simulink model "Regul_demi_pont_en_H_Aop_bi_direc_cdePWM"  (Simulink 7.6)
settings: Solver=ode15s  StartTime=0.0  StopTime=0.01  FixedStep=0.01  RelTol=1e-3
InitFcn:
  | clc
  | delete *.mat
  | close all
  | clear all
StopFcn:
  | close all, clc
  | load reg_vit.mat
  | 
  | plot(x(1,:),x(2,:),x(1,:),x(3,:))
  | xlabel('temps')
  | title('Consigne et vitesse angulaire - Moteur CC, 1/2 Pont en H bidirectionnel - Cde PWM')
  | grid
  | 
  | figure
  | load cde_PWM.mat
  | plot(u(1,:),u(2,:))
  | axis([0 4e-3 -0.5 5.5])
  | xlabel('temps')
  | title('Commande PWM')
  | grid
undefined symbols (not defined in the file or in its folder): sigbuilder_block
libraries: fl_lib x24, elec_lib x15, nesl_utility x15, simulink x1

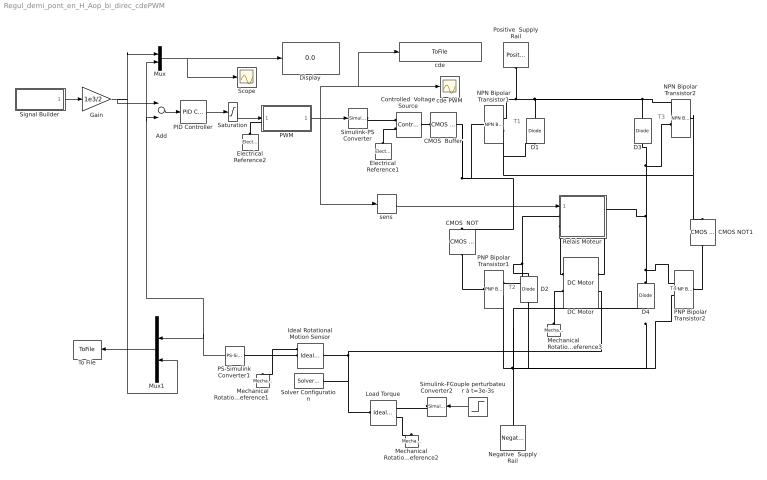
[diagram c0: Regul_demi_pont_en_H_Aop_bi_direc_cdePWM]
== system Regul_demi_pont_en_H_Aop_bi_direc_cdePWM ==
  note: T1
  note: T4
  note: T3
  note: T2
  Add : Sum  Inputs=+-
  CMOS  Buffer : elec_lib/Integrated Circuits/Logic/CMOS Buffer  DialogController=NetworkEngine.DynNeDlgSource  SystemSampleTime=-1  V_IL=2 V  V_IH=3 V  C_IN=5 pF  output_type=1  V_OL=0 V  V_OH=5 V  V_CC=5 V  V_meas=5 V  R_OUT=25 Ohm  R_OH=[ 25 250 ] Ohm  I_OH=63 mA  R_OL=[ 30 800 ] Ohm  I_OL=-45 mA  Delay=25 ns  Ron=5 Ohm  Vf=0.6 V  output_state=1  LocalVarLogging=[]
  CMOS  NOT : elec_lib/Integrated Circuits/Logic/CMOS NOT  DialogController=NetworkEngine.DynNeDlgSource  SystemSampleTime=-1  V_IL=2 V  V_IH=3 V  C_IN=5 pF  output_type=1  V_OL=0 V  V_OH=5 V  V_CC=5 V  V_meas=5 V  R_OUT=25 Ohm  R_OH=[ 25 250 ] Ohm  I_OH=63 mA  R_OL=[ 30 800 ] Ohm  I_OL=-45 mA  Delay=25 ns  Ron=5 Ohm  Vf=0.6 V  output_state=1  LocalVarLogging=[]
  CMOS NOT1 : elec_lib/Integrated Circuits/Logic/CMOS NOT  DialogController=NetworkEngine.DynNeDlgSource  SystemSampleTime=-1  V_IL=2 V  V_IH=3 V  C_IN=5 pF  output_type=1  V_OL=0 V  V_OH=5 V  V_CC=5 V  V_meas=5 V  R_OUT=25 Ohm  R_OH=[ 25 250 ] Ohm  I_OH=63 mA  R_OL=[ 30 800 ] Ohm  I_OL=-45 mA  Delay=25 ns  Ron=5 Ohm  Vf=0.6 V  output_state=1  LocalVarLogging=[]
  Controlled  Voltage Source : fl_lib/Electrical/Electrical Sources/Controlled Voltage Source  DialogController=NetworkEngine.DynNeDlgSource  SystemSampleTime=-1  i_Log=off  v_Log=off  LocalVarNames=|i|v  LocalVarDescs=|i|v  LocalVarLogging=[0 0]
  Couple perturbateur à t=3e-3s : Step  Time=0.001  After=-4e-3  SampleTime=0
  D{1..4} (4 alike) : elec_lib/Semiconductor Devices/Diode  DialogController=NetworkEngine.DynNeDlgSource  SystemSampleTime=-1  ModelType=1  Vf=0.6 V  Ron=0.3 Ohm  Goff=1e-8 S  Rz=0.3 Ohm  Vz=50 V  C_PWL=5 pF  prmExp=1  I12=[ 0.07 1.5 ] A  V12=[ 0.7 0.8 ] V  I1=0.07 A  V1=0.7 V  RS=0.01 Ohm  IS=1e-14 A  Tmeas=25 C  ec=1  BV=Inf V  C_param=1  CJ0=5 pF  VJ=1 V  Mgrad=0.5  Vvec=[ 0.1 10 100 ] V  Cvec=[ 3.5 1 0.4 ] pF  FC=0.5  LocalVarLogging=[]
  DC Motor : elec_lib/Actuators & Drivers/Rotational Actuators/DC Motor  DialogController=NetworkEngine.DynNeDlgSource  SystemSampleTime=-1  parameterization=1  Ra=3.9 Ohm  La=1.2e-5 H  emf_or_torque=1  Kv=7.2e-5 V/rpm  Ki=6.876e-4 N*m/A  T_stall=2.4e-4 N*m  w_max=1.91e+4 rpm  w_rated=1.5e+4 rpm  P_rated=0.08 W  V_rated=1.5 V  J=0.01 g*cm^2  lam=1e-8 N*m/(rad/s)  speed0=0.5 rpm  current_Log=off  voltage_Log=off  power_Log=off  i2r_Log=off  torque_Log=off  speed_Log=off  LocalVarNames=|current|voltage|power|i2r|torque|speed  LocalVarDescs=|Current (A)|Voltage (V)|Power (W)|Electrical losses (W)|Torque (Nm)|Angular speed (rad/s)  LocalVarLogging=[0 0 0 0 0 0]
  Display : Display
  Electrical Reference1 : fl_lib/Electrical/Electrical Elements/Electrical Reference  DialogController=NetworkEngine.DynNeDlgSource  SystemSampleTime=-1  i_Log=off  LocalVarNames=|i  LocalVarDescs=|i  LocalVarLogging=[]
  Electrical Reference2 : fl_lib/Electrical/Electrical Elements/Electrical Reference  DialogController=NetworkEngine.DynNeDlgSource  SystemSampleTime=-1  i_Log=off  LocalVarNames=|i  LocalVarDescs=|i  LocalVarLogging=[]
  Gain : Gain  Gain=1e3/2
  Ideal Rotational Motion Sensor : fl_lib/Mechanical/Mechanical Sensors/Ideal Rotational Motion Sensor  DialogController=NetworkEngine.DynNeDlgSource  SystemSampleTime=-1  offset=0 rad  w_Log=off  t_Log=off  phi_Log=off  LocalVarNames=|w|t|phi  LocalVarDescs=|w|t|phi  LocalVarLogging=[0 0 0]
  Load Torque : fl_lib/Mechanical/Mechanical Sources/Ideal Torque Source  DialogController=NetworkEngine.DynNeDlgSource  SystemSampleTime=-1  w_Log=off  t_Log=off  LocalVarNames=|torque|rel_velocity|power  LocalVarDescs=|Torque (N*m)|Relative velocity (rad/s)|Power generated by the source (W)  LocalVarLogging=[0 0 0]
  Mechanical Rotational Reference1 : fl_lib/Mechanical/Rotational Elements/Mechanical Rotational Reference  DialogController=NetworkEngine.DynNeDlgSource  SystemSampleTime=-1  t_Log=off  LocalVarNames=|t  LocalVarDescs=|t  LocalVarLogging=0
  Mechanical Rotational Reference2 : fl_lib/Mechanical/Rotational Elements/Mechanical Rotational Reference  DialogController=NetworkEngine.DynNeDlgSource  SystemSampleTime=-1  t_Log=off  LocalVarNames=|t  LocalVarDescs=|t  LocalVarLogging=[]
  Mechanical Rotational Reference3 : fl_lib/Mechanical/Rotational Elements/Mechanical Rotational Reference  DialogController=NetworkEngine.DynNeDlgSource  SystemSampleTime=-1  t_Log=off  LocalVarNames=|t  LocalVarDescs=|t  LocalVarLogging=0
  Mux : Mux  Inputs=2
  Mux1 : Mux  Inputs=2
  NPN Bipolar Transistor1 : elec_lib/Semiconductor Devices/NPN Bipolar Transistor  DialogController=NetworkEngine.DynNeDlgSource  SystemSampleTime=-1  parameterization=1  BF=100  IS=1e-14 A  VAF=200 V  hfe=100  hoe=5e-5 1/Ohm  Ic_h=1 mA  V1=0.55 V  I1=0.5 mA  BR=1  Tmeas=25 C  RC=0.01 Ohm  RE=1e-4 Ohm  RB=1 Ohm  C_BC=5 pF  C_BE=5 pF  TF=0 us  TR=0 us  LocalVarLogging=[]
  NPN Bipolar Transistor2 : elec_lib/Semiconductor Devices/NPN Bipolar Transistor  DialogController=NetworkEngine.DynNeDlgSource  SystemSampleTime=-1  parameterization=1  BF=100  IS=1e-14 A  VAF=200 V  hfe=100  hoe=5e-5 1/Ohm  Ic_h=1 mA  V1=0.55 V  I1=0.5 mA  BR=1  Tmeas=25 C  RC=0.01 Ohm  RE=1e-4 Ohm  RB=1 Ohm  C_BC=5 pF  C_BE=5 pF  TF=0 us  TR=0 us  LocalVarLogging=[]
  Negative  Supply Rail : elec_lib/Sources/Negative Supply Rail  DialogController=NetworkEngine.DynNeDlgSource  SystemSampleTime=-1  v0=-24 V  current_Log=off  voltage_Log=off  power_Log=off  LocalVarNames=|current|voltage|power  LocalVarDescs=|Current (A)|Voltage (V)|Power (W)  LocalVarLogging=[0 0 0]
  PID Controller : simulink/Continuous/PID Controller  DialogController=pidpack.PIDConfig.pidDDGCreate  DialogControllerArgs=DataTag0  SystemSampleTime=-1  Controller=PID  TimeDomain=Continuous-time  SampleTime=1  IntegratorMethod=Forward Euler  FilterMethod=Forward Euler  Form=Parallel  P=10  I=0.1  D=0  N=100  InitialConditionSource=internal  InitialConditionForIntegrator=0  InitialConditionForFilter=0  ExternalReset=none  LimitOutput=off  UpperSaturationLimit=inf  LowerSaturationLimit=-inf  LinearizeAsGain=off  AntiWindupMode=none  Kb=1  TrackingMode=off  Kt=1  PParamMin=[]  PParamMax=[]  IParamMin=[]  IParamMax=[]  DParamMin=[]  DParamMax=[]  NParamMin=[]  NParamMax=[]  KbParamMin=[]  KbParamMax=[]  KtParamMin=[]  KtParamMax=[]  POutMin=[]  POutMax=[]  IOutMin=[]  IOutMax=[]  DOutMin=[]  DOutMax=[]  NOutMin=[]  NOutMax=[]  KbOutMin=[]  KbOutMax=[]  KtOutMin=[]  KtOutMax=[]  IntegratorOutMin=[]  IntegratorOutMax=[]  FilterOutMin=[]  FilterOutMax=[]  SumOutMin=[]  SumOutMax=[]  SumI1OutMin=[]  SumI1OutMax=[]  SumI2OutMin=[]  SumI2OutMax=[]  SumI3OutMin=[]  SumI3OutMax=[]  SumDOutMin=[]  SumDOutMax=[]  SaturationOutMin=[]  SaturationOutMax=[]  IntegratorContinuousStateAttributes=''  IntegratorStateMustResolveToSignalObject=off  IntegratorRTWStateStorageClass=Auto  FilterContinuousStateAttributes=''  FilterStateMustResolveToSignalObject=off  FilterRTWStateStorageClass=Auto
  PNP Bipolar Transistor1 : elec_lib/Semiconductor Devices/PNP Bipolar Transistor  DialogController=NetworkEngine.DynNeDlgSource  SystemSampleTime=-1  parameterization=1  BF=100  IS=1e-14 A  VAF=200 V  hfe=100  hoe=5e-5 1/Ohm  Ic_h=1 mA  V1=0.55 V  I1=0.5 mA  BR=1  Tmeas=25 C  RC=0.01 Ohm  RE=1e-4 Ohm  RB=1 Ohm  C_BC=5 pF  C_BE=5 pF  TF=0 us  TR=0 us  LocalVarLogging=[]
  PNP Bipolar Transistor2 : elec_lib/Semiconductor Devices/PNP Bipolar Transistor  DialogController=NetworkEngine.DynNeDlgSource  SystemSampleTime=-1  parameterization=1  BF=100  IS=1e-14 A  VAF=200 V  hfe=100  hoe=5e-5 1/Ohm  Ic_h=1 mA  V1=0.55 V  I1=0.5 mA  BR=1  Tmeas=25 C  RC=0.01 Ohm  RE=1e-4 Ohm  RB=1 Ohm  C_BC=5 pF  C_BE=5 pF  TF=0 us  TR=0 us  LocalVarLogging=[]
  PS-Simulink Converter1 : nesl_utility/PS-Simulink Converter  DialogController=NetworkEngine.DynNeUtilDlgSource  SystemSampleTime=-1  PhysicalDomain=network_engine_domain  LeftPortType=input  RightPortType=output  SubClassName=ps_output  Unit=1  AffineConversion=off
  PWM : Subsystem
  Positive  Supply Rail : elec_lib/Sources/Positive Supply Rail  DialogController=NetworkEngine.DynNeDlgSource  SystemSampleTime=-1  v0=24 V  current_Log=off  voltage_Log=off  power_Log=off  LocalVarNames=|current|voltage|power  LocalVarDescs=|Current (A)|Voltage (V)|Power (W)  LocalVarLogging=[0 0 0]
  Relais Moteur : Subsystem
  Saturation : Saturate  UpperLimit=5  LowerLimit=0
  Scope : Scope
  Signal Builder : Subsystem  Tag=STV Subsys  LoadFcn=sigbuilder_block('load');  StartFcn=sigbuilder_block('start');  StopFcn=sigbuilder_block('stop');  ClipboardFcn=sigbuilder_block('clipboard');
  Simulink-PS Converter : nesl_utility/Simulink-PS Converter  DialogController=NetworkEngine.DynNeUtilDlgSource  SystemSampleTime=-1  PhysicalDomain=network_engine_domain  LeftPortType=input  RightPortType=output  SubClassName=ps_input  Unit=1  AffineConversion=off  InputFilterTimeConstant=.001  UdotUserProvided=0
  Simulink-PS Converter2 : nesl_utility/Simulink-PS Converter  DialogController=NetworkEngine.DynNeUtilDlgSource  SystemSampleTime=-1  PhysicalDomain=network_engine_domain  LeftPortType=input  RightPortType=output  SubClassName=ps_input  Unit=1  AffineConversion=off  InputFilterTimeConstant=.001  UdotUserProvided=0
  Solver Configuration : nesl_utility/Solver Configuration  DialogController=NetworkEngine.DynNeUtilDlgSource  SystemSampleTime=-1  PhysicalDomain=network_engine_domain  LeftPortType=input  RightPortType=generic  SubClassName=solver  Accelerate=off  Profile=off  ResidualTolerance=1e-9  MaxNonlinIter=3  MaxModeIter=2  DoFixedCost=off  UseLocalSampling=off  DoDC=off  LinearAlgebra=Sparse  LocalSolverSampleTime=.001  LocalSolverChoice=NE_BACKWARD_EULER_ADVANCER  UseLocalSolver=off
  To File : ToFile  Filename=reg_vit  MatrixName=x
  cde : ToFile  Filename=cde_PWM  MatrixName=u
  cde PWM : Scope
  sens : Signum
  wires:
  Mux1/1 -> To File/1
  PWM/1(PWM) -> Simulink-PS Converter/1, sens/1, cde PWM/1, cde/1
  PS-Simulink Converter1/1 -> Mux1/1, Add/2, Mux/2
  Gain/1 -> Add/1, Mux/1, Mux1/2
  Signal Builder/1(Signal 2) -> Gain/1
  PID Controller/1 -> Saturation/1
  Add/1 -> PID Controller/1
  Mux/1 -> Display/1, Scope/1
  Saturation/1 -> PWM/1(+ref)
  Couple perturbateur à t=3e-3s/1 -> Simulink-PS Converter2/1
  sens/1 -> Relais Moteur/1(cde_sens)
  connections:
  D3/RConn1 -- NPN Bipolar Transistor2/RConn1 -- Positive  Supply Rail/RConn1 -- NPN Bipolar Transistor1/RConn1 -- D1/RConn1
  CMOS  Buffer/LConn1 -- Controlled  Voltage Source/LConn1
  Simulink-PS Converter/RConn1 -- Controlled  Voltage Source/RConn1
  Relais Moteur/LConn1 -- PNP Bipolar Transistor1/RConn1 -- D2/RConn1
  D4/RConn1 -- PNP Bipolar Transistor2/RConn1 -- Relais Moteur/RConn1 -- D3/LConn1 -- NPN Bipolar Transistor2/RConn2
  Relais Moteur/LConn2 -- DC Motor/RConn1
  Relais Moteur/RConn2 -- DC Motor/LConn1
  Mechanical Rotational Reference3/LConn1 -- DC Motor/RConn2
  D4/LConn1 -- PNP Bipolar Transistor2/RConn2 -- PNP Bipolar Transistor1/RConn2 -- D2/LConn1 -- Negative  Supply Rail/LConn1
  Solver Configuration/RConn1 -- DC Motor/LConn2 -- Ideal Rotational Motion Sensor/LConn1 -- Load Torque/LConn1
  NPN Bipolar Transistor1/RConn2 -- NPN Bipolar Transistor1/LConn1 -- CMOS  Buffer/RConn1 -- CMOS  NOT/LConn1 -- CMOS NOT1/LConn1 -- NPN Bipolar Transistor2/LConn1 -- D1/LConn1
  CMOS  NOT/RConn1 -- PNP Bipolar Transistor1/LConn1
  CMOS NOT1/RConn1 -- PNP Bipolar Transistor2/LConn1
  Electrical Reference2/LConn1 -- PWM/LConn1
  Ideal Rotational Motion Sensor/RConn2 -- PS-Simulink Converter1/LConn1
  Electrical Reference1/LConn1 -- Controlled  Voltage Source/RConn2
  Load Torque/RConn2 -- Mechanical Rotational Reference2/LConn1
  Simulink-PS Converter2/RConn1 -- Load Torque/RConn1
  Ideal Rotational Motion Sensor/RConn1 -- Mechanical Rotational Reference1/LConn1

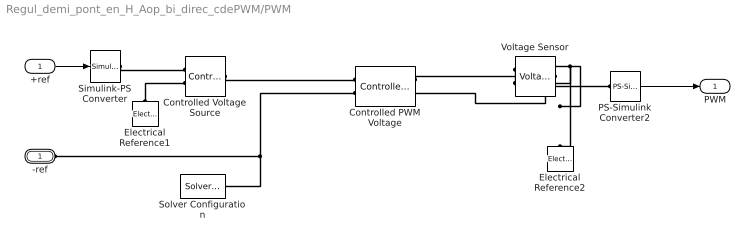
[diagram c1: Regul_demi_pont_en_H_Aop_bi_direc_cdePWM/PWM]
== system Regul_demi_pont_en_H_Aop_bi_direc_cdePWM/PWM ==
  +ref : Inport
  Controlled PWM Voltage : elec_lib/Actuators & Drivers/Drivers/Controlled PWM Voltage  DialogController=NetworkEngine.DynNeDlgSource  SystemSampleTime=-1  F=10000 Hz  Vmin=0 V  Vmax=5 V  Vm=5 V  pwm_or_av=1  current_Log=off  voltage_Log=off  power_Log=off  LocalVarNames=|current|voltage|power  LocalVarDescs=|Load current (A)|Load voltage (V)|Load power (W)  LocalVarLogging=[0 0 0]
  Controlled Voltage Source : fl_lib/Electrical/Electrical Sources/Controlled Voltage Source  DialogController=NetworkEngine.DynNeDlgSource  SystemSampleTime=-1  i_Log=off  v_Log=off  LocalVarNames=|i|v  LocalVarDescs=|i|v  LocalVarLogging=[0 0]
  Electrical Reference1 : fl_lib/Electrical/Electrical Elements/Electrical Reference  DialogController=NetworkEngine.DynNeDlgSource  SystemSampleTime=-1  i_Log=off  LocalVarNames=|i  LocalVarDescs=|i  LocalVarLogging=[]
  Electrical Reference2 : fl_lib/Electrical/Electrical Elements/Electrical Reference  DialogController=NetworkEngine.DynNeDlgSource  SystemSampleTime=-1  i_Log=off  LocalVarNames=|i  LocalVarDescs=|i  LocalVarLogging=[]
  PS-Simulink Converter2 : nesl_utility/PS-Simulink Converter  DialogController=NetworkEngine.DynNeUtilDlgSource  SystemSampleTime=-1  PhysicalDomain=network_engine_domain  LeftPortType=input  RightPortType=output  SubClassName=ps_output  Unit=1  AffineConversion=off
  Simulink-PS Converter : nesl_utility/Simulink-PS Converter  DialogController=NetworkEngine.DynNeUtilDlgSource  SystemSampleTime=-1  PhysicalDomain=network_engine_domain  LeftPortType=input  RightPortType=output  SubClassName=ps_input  Unit=1  AffineConversion=off  InputFilterTimeConstant=.001  UdotUserProvided=0
  Solver Configuration : nesl_utility/Solver Configuration  DialogController=NetworkEngine.DynNeUtilDlgSource  SystemSampleTime=-1  PhysicalDomain=network_engine_domain  LeftPortType=input  RightPortType=generic  SubClassName=solver  Accelerate=off  Profile=off  ResidualTolerance=1e-9  MaxNonlinIter=3  MaxModeIter=2  DoFixedCost=off  UseLocalSampling=off  DoDC=off  LinearAlgebra=Sparse  LocalSolverSampleTime=.001  LocalSolverChoice=NE_BACKWARD_EULER_ADVANCER  UseLocalSolver=off
  Voltage Sensor : fl_lib/Electrical/Electrical Sensors/Voltage Sensor  DialogController=NetworkEngine.DynNeDlgSource  SystemSampleTime=-1  i1_Log=off  v1_Log=off  LocalVarNames=|i1|v1  LocalVarDescs=|i1|v1  LocalVarLogging=[0 0]
  -ref : PMIOPort  Port=1  Side=Left
  PWM : Outport
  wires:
  PS-Simulink Converter2/1 -> PWM/1
  +ref/1 -> Simulink-PS Converter/1
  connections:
  -ref/RConn1 -- Controlled PWM Voltage/LConn2 -- Solver Configuration/RConn1
  Controlled PWM Voltage/RConn1 -- Voltage Sensor/LConn1
  Voltage Sensor/RConn2 -- Controlled PWM Voltage/RConn2 -- Electrical Reference2/LConn1
  Voltage Sensor/RConn1 -- PS-Simulink Converter2/LConn1
  Controlled Voltage Source/LConn1 -- Controlled PWM Voltage/LConn1
  Electrical Reference1/LConn1 -- Controlled Voltage Source/RConn2
  Simulink-PS Converter/RConn1 -- Controlled Voltage Source/RConn1

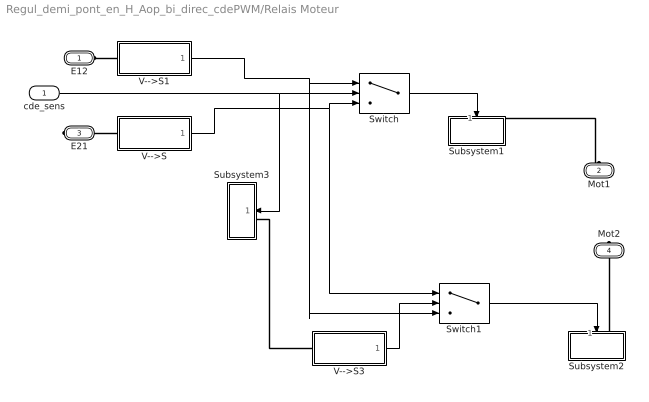
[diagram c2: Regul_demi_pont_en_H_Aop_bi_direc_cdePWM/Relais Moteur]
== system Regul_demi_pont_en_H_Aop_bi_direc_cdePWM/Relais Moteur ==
  cde_sens : Inport
  Subsystem1 : Subsystem
  Subsystem2 : Subsystem
  Subsystem3 : Subsystem
  Switch : Switch  Threshold=0.5
  Switch1 : Switch  Threshold=0.5
  V-->S : Subsystem
  V-->S1 : Subsystem
  V-->S3 : Subsystem
  E12 : PMIOPort  Port=1  Side=Left
  Mot1 : PMIOPort  Port=2  Side=Left
  E21 : PMIOPort  Port=3  Side=Right
  Mot2 : PMIOPort  Port=4  Side=Right
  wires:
  V-->S/1(S) -> Switch/3, Switch1/1
  V-->S1/1(S) -> Switch/1, Switch1/3
  V-->S3/1(S) -> Switch1/2
  Switch/1 -> Subsystem1/1(S)
  cde_sens/1 -> Switch/2, Subsystem3/1(S)
  Switch1/1 -> Subsystem2/1(S)
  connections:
  Subsystem1/LConn1 -- Mot1/RConn1
  Subsystem3/LConn1 -- V-->S3/LConn1
  E12/RConn1 -- V-->S1/LConn1
  E21/RConn1 -- V-->S/LConn1
  Mot2/RConn1 -- Subsystem2/LConn1

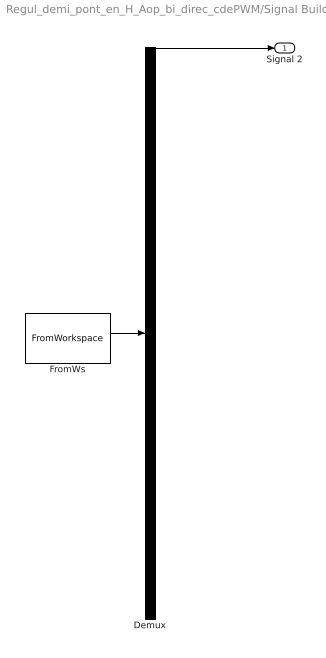
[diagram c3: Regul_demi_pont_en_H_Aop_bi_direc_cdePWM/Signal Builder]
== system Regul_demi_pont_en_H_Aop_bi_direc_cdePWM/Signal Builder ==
  Demux : Demux  Tag=STV Demux  Outputs=1
  FromWs : FromWorkspace  Tag=STV FromWs  VariableName=tuvar  SampleTime=0  SigBuilderData=DataTag1  VnvData=DataTag2
  Signal 2 : Outport  Tag=STV Outport
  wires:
  FromWs/1 -> Demux/1
  Demux/1 -> Signal 2/1

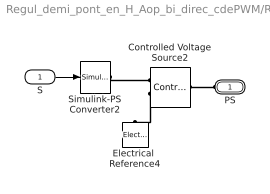
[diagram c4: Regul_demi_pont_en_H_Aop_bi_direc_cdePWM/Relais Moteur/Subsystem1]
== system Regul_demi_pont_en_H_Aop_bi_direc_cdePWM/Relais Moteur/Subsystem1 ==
  S : Inport
  Controlled Voltage Source2 : fl_lib/Electrical/Electrical Sources/Controlled Voltage Source  DialogController=NetworkEngine.DynNeDlgSource  SystemSampleTime=-1  i_Log=off  v_Log=off  LocalVarNames=|i|v  LocalVarDescs=|i|v  LocalVarLogging=[0 0]
  Electrical  Reference4 : fl_lib/Electrical/Electrical Elements/Electrical Reference  DialogController=NetworkEngine.DynNeDlgSource  SystemSampleTime=-1  i_Log=off  LocalVarNames=|i  LocalVarDescs=|i  LocalVarLogging=0
  Simulink-PS Converter2 : nesl_utility/Simulink-PS Converter  DialogController=NetworkEngine.DynNeUtilDlgSource  SystemSampleTime=-1  PhysicalDomain=network_engine_domain  LeftPortType=input  RightPortType=output  SubClassName=ps_input  Unit=1  AffineConversion=off  InputFilterTimeConstant=.001  UdotUserProvided=0
  PS : PMIOPort  Port=1  Side=Left
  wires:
  S/1 -> Simulink-PS Converter2/1
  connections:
  PS/RConn1 -- Controlled Voltage Source2/LConn1
  Controlled Voltage Source2/RConn2 -- Electrical  Reference4/LConn1
  Simulink-PS Converter2/RConn1 -- Controlled Voltage Source2/RConn1

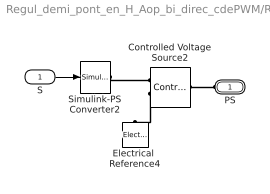
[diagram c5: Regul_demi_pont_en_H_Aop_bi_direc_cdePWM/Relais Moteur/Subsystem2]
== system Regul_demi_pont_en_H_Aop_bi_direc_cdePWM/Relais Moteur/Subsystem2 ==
  S : Inport
  Controlled Voltage Source2 : fl_lib/Electrical/Electrical Sources/Controlled Voltage Source  DialogController=NetworkEngine.DynNeDlgSource  SystemSampleTime=-1  i_Log=off  v_Log=off  LocalVarNames=|i|v  LocalVarDescs=|i|v  LocalVarLogging=[0 0]
  Electrical  Reference4 : fl_lib/Electrical/Electrical Elements/Electrical Reference  DialogController=NetworkEngine.DynNeDlgSource  SystemSampleTime=-1  i_Log=off  LocalVarNames=|i  LocalVarDescs=|i  LocalVarLogging=0
  Simulink-PS Converter2 : nesl_utility/Simulink-PS Converter  DialogController=NetworkEngine.DynNeUtilDlgSource  SystemSampleTime=-1  PhysicalDomain=network_engine_domain  LeftPortType=input  RightPortType=output  SubClassName=ps_input  Unit=1  AffineConversion=off  InputFilterTimeConstant=.001  UdotUserProvided=0
  PS : PMIOPort  Port=1  Side=Left
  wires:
  S/1 -> Simulink-PS Converter2/1
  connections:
  Simulink-PS Converter2/RConn1 -- Controlled Voltage Source2/RConn1
  Controlled Voltage Source2/RConn2 -- Electrical  Reference4/LConn1
  PS/RConn1 -- Controlled Voltage Source2/LConn1

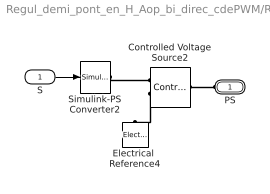
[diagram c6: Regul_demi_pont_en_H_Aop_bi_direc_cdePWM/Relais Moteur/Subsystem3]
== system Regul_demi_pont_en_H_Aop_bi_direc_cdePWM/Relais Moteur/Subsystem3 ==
  S : Inport
  Controlled Voltage Source2 : fl_lib/Electrical/Electrical Sources/Controlled Voltage Source  DialogController=NetworkEngine.DynNeDlgSource  SystemSampleTime=-1  i_Log=off  v_Log=off  LocalVarNames=|i|v  LocalVarDescs=|i|v  LocalVarLogging=[0 0]
  Electrical  Reference4 : fl_lib/Electrical/Electrical Elements/Electrical Reference  DialogController=NetworkEngine.DynNeDlgSource  SystemSampleTime=-1  i_Log=off  LocalVarNames=|i  LocalVarDescs=|i  LocalVarLogging=0
  Simulink-PS Converter2 : nesl_utility/Simulink-PS Converter  DialogController=NetworkEngine.DynNeUtilDlgSource  SystemSampleTime=-1  PhysicalDomain=network_engine_domain  LeftPortType=input  RightPortType=output  SubClassName=ps_input  Unit=1  AffineConversion=off  InputFilterTimeConstant=.001  UdotUserProvided=0
  PS : PMIOPort  Port=1  Side=Left
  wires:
  S/1 -> Simulink-PS Converter2/1
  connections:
  PS/RConn1 -- Controlled Voltage Source2/LConn1
  Controlled Voltage Source2/RConn2 -- Electrical  Reference4/LConn1
  Simulink-PS Converter2/RConn1 -- Controlled Voltage Source2/RConn1

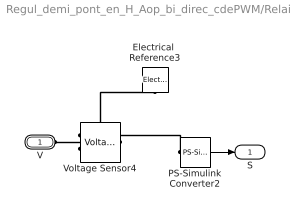
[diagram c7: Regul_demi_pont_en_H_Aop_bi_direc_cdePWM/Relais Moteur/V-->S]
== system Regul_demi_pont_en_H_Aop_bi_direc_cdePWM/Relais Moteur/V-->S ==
  Electrical  Reference3 : fl_lib/Electrical/Electrical Elements/Electrical Reference  DialogController=NetworkEngine.DynNeDlgSource  SystemSampleTime=-1  i_Log=off  LocalVarNames=|i  LocalVarDescs=|i  LocalVarLogging=0
  PS-Simulink Converter2 : nesl_utility/PS-Simulink Converter  DialogController=NetworkEngine.DynNeUtilDlgSource  SystemSampleTime=-1  PhysicalDomain=network_engine_domain  LeftPortType=input  RightPortType=output  SubClassName=ps_output  Unit=1  AffineConversion=off
  Voltage Sensor4 : fl_lib/Electrical/Electrical Sensors/Voltage Sensor  DialogController=NetworkEngine.DynNeDlgSource  SystemSampleTime=-1  i1_Log=off  v1_Log=off  LocalVarNames=|i1|v1  LocalVarDescs=|i1|v1  LocalVarLogging=[0 0]
  V : PMIOPort  Port=1  Side=Left
  S : Outport
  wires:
  PS-Simulink Converter2/1 -> S/1
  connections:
  Voltage Sensor4/RConn2 -- Electrical  Reference3/LConn1
  PS-Simulink Converter2/LConn1 -- Voltage Sensor4/RConn1
  V/RConn1 -- Voltage Sensor4/LConn1

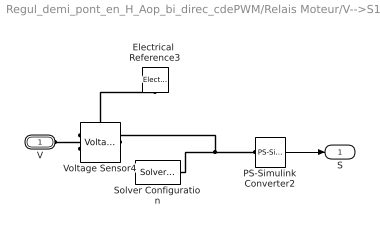
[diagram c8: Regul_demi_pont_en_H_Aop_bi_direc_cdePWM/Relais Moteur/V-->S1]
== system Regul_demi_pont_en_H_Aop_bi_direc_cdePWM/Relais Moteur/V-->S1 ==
  Electrical  Reference3 : fl_lib/Electrical/Electrical Elements/Electrical Reference  DialogController=NetworkEngine.DynNeDlgSource  SystemSampleTime=-1  i_Log=off  LocalVarNames=|i  LocalVarDescs=|i  LocalVarLogging=0
  PS-Simulink Converter2 : nesl_utility/PS-Simulink Converter  DialogController=NetworkEngine.DynNeUtilDlgSource  SystemSampleTime=-1  PhysicalDomain=network_engine_domain  LeftPortType=input  RightPortType=output  SubClassName=ps_output  Unit=1  AffineConversion=off
  Solver Configuration : nesl_utility/Solver Configuration  DialogController=NetworkEngine.DynNeUtilDlgSource  SystemSampleTime=-1  PhysicalDomain=network_engine_domain  LeftPortType=input  RightPortType=generic  SubClassName=solver  Accelerate=off  Profile=off  ResidualTolerance=1e-9  MaxNonlinIter=3  MaxModeIter=2  DoFixedCost=off  UseLocalSampling=off  DoDC=off  LinearAlgebra=Sparse  LocalSolverSampleTime=.001  LocalSolverChoice=NE_BACKWARD_EULER_ADVANCER  UseLocalSolver=off
  Voltage Sensor4 : fl_lib/Electrical/Electrical Sensors/Voltage Sensor  DialogController=NetworkEngine.DynNeDlgSource  SystemSampleTime=-1  i1_Log=off  v1_Log=off  LocalVarNames=|i1|v1  LocalVarDescs=|i1|v1  LocalVarLogging=[0 0]
  V : PMIOPort  Port=1  Side=Left
  S : Outport
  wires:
  PS-Simulink Converter2/1 -> S/1
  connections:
  V/RConn1 -- Voltage Sensor4/LConn1
  PS-Simulink Converter2/LConn1 -- Voltage Sensor4/RConn1 -- Solver Configuration/RConn1
  Voltage Sensor4/RConn2 -- Electrical  Reference3/LConn1

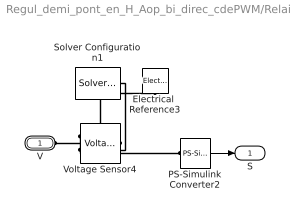
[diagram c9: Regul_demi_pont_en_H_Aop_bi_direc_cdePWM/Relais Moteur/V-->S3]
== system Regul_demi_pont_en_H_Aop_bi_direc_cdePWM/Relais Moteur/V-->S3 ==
  Electrical  Reference3 : fl_lib/Electrical/Electrical Elements/Electrical Reference  DialogController=NetworkEngine.DynNeDlgSource  SystemSampleTime=-1  i_Log=off  LocalVarNames=|i  LocalVarDescs=|i  LocalVarLogging=0
  PS-Simulink Converter2 : nesl_utility/PS-Simulink Converter  DialogController=NetworkEngine.DynNeUtilDlgSource  SystemSampleTime=-1  PhysicalDomain=network_engine_domain  LeftPortType=input  RightPortType=output  SubClassName=ps_output  Unit=1  AffineConversion=off
  Solver Configuration1 : nesl_utility/Solver Configuration  DialogController=NetworkEngine.DynNeUtilDlgSource  SystemSampleTime=-1  PhysicalDomain=network_engine_domain  LeftPortType=input  RightPortType=generic  SubClassName=solver  Accelerate=off  Profile=off  ResidualTolerance=1e-9  MaxNonlinIter=3  MaxModeIter=2  DoFixedCost=off  UseLocalSampling=off  DoDC=off  LinearAlgebra=Sparse  LocalSolverSampleTime=.001  LocalSolverChoice=NE_BACKWARD_EULER_ADVANCER  UseLocalSolver=off
  Voltage Sensor4 : fl_lib/Electrical/Electrical Sensors/Voltage Sensor  DialogController=NetworkEngine.DynNeDlgSource  SystemSampleTime=-1  i1_Log=off  v1_Log=off  LocalVarNames=|i1|v1  LocalVarDescs=|i1|v1  LocalVarLogging=[0 0]
  V : PMIOPort  Port=1  Side=Left
  S : Outport
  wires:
  PS-Simulink Converter2/1 -> S/1
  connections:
  Voltage Sensor4/RConn2 -- Electrical  Reference3/LConn1 -- Solver Configuration1/RConn1
  Voltage Sensor4/RConn1 -- PS-Simulink Converter2/LConn1
  V/RConn1 -- Voltage Sensor4/LConn1
